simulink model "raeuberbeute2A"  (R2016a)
settings: Solver=ode45  StartTime=0.0  StopTime=250  FixedStep=0.1  MaxStep=1  RelTol=1e-3
undefined symbols (not defined in the file or in its folder): k, m0
libraries: simulink x1

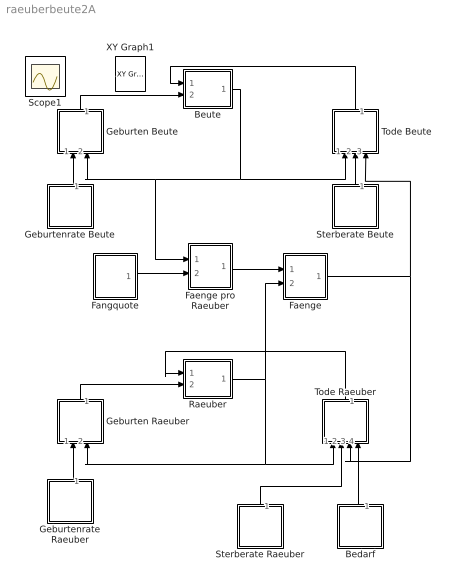
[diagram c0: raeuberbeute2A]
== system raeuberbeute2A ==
  Bedarf : Subsystem
  Beute : Subsystem
  Faenge : Subsystem
  Faenge pro Raeuber : Subsystem
  Fangquote : Subsystem
  Geburten Beute : Subsystem
  Geburten Raeuber : Subsystem
  Geburtenrate Beute : Subsystem
  Geburtenrate Raeuber : Subsystem
  Raeuber : Subsystem
  Sterberate Beute : Subsystem
  Sterberate Raeuber : Subsystem
  Tode Beute : Subsystem
  Tode Raeuber : Subsystem
  Scope1 : Scope
  XY Graph1 : simulink/Sinks/XY Graph  IOType=viewer  SystemSampleTime=-1  xmin=0  xmax=30  ymin=0  ymax=60  st=-1
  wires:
  Beute/1(Out1) -> Tode Beute/1(In1), Geburten Beute/2(In2), Faenge pro Raeuber/1(In1)
  Faenge/1(Out1) -> Tode Beute/3(In3), Tode Raeuber/3(In3)
  Raeuber/1(Out1) -> Geburten Raeuber/2(In2), Tode Raeuber/1(In1), Faenge/2(In2)
  Fangquote/1(Out1) -> Faenge pro Raeuber/2(In2)
  Geburten Beute/1(Out1) -> Beute/2(In2)
  Geburtenrate Beute/1(Out1) -> Geburten Beute/1(In1)
  Tode Beute/1(Out1) -> Beute/1(In1)
  Sterberate Beute/1(Out1) -> Tode Beute/2(In2)
  Geburten Raeuber/1(Out1) -> Raeuber/2(In2)
  Geburtenrate Raeuber/1(Out1) -> Geburten Raeuber/1(In1)
  Tode Raeuber/1(Out1) -> Raeuber/1(In1)
  Bedarf/1(Out1) -> Tode Raeuber/4(In4)
  Sterberate Raeuber/1(Out1) -> Tode Raeuber/2(In2)
  Faenge pro Raeuber/1(Out1) -> Faenge/1(In1)

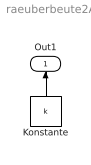
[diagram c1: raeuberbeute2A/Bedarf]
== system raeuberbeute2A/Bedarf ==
  Konstante : Constant  Value=k
  Out1 : Outport
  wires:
  Konstante/1 -> Out1/1

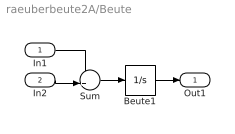
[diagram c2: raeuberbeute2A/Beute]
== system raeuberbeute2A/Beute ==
  In1 : Inport
  In2 : Inport  Port=2
  Beute1 : Integrator  InitialCondition=m0
  Sum : Sum  Inputs=-+|
  Out1 : Outport
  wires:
  In2/1 -> Sum/2
  Beute1/1 -> Out1/1
  In1/1 -> Sum/1
  Sum/1 -> Beute1/1

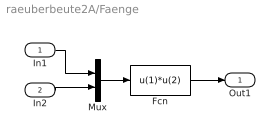
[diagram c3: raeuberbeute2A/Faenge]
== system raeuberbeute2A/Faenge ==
  In1 : Inport
  In2 : Inport  Port=2
  Fcn : Fcn  Expr=u(1)*u(2)
  Mux : Mux  Inputs=2
  Out1 : Outport
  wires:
  In2/1 -> Mux/2
  In1/1 -> Mux/1
  Mux/1 -> Fcn/1
  Fcn/1 -> Out1/1

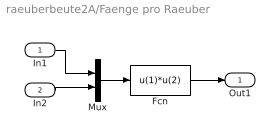
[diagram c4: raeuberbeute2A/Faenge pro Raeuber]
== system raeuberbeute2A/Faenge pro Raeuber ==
  In1 : Inport
  In2 : Inport  Port=2
  Fcn : Fcn  Expr=u(1)*u(2)
  Mux : Mux  Inputs=2
  Out1 : Outport
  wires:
  In2/1 -> Mux/2
  In1/1 -> Mux/1
  Mux/1 -> Fcn/1
  Fcn/1 -> Out1/1

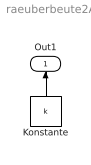
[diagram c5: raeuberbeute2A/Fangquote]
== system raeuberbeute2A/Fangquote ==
  Konstante : Constant  Value=k
  Out1 : Outport
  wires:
  Konstante/1 -> Out1/1

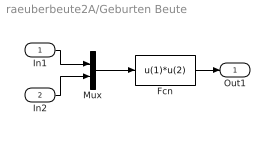
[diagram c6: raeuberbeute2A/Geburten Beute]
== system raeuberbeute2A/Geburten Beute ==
  In1 : Inport
  In2 : Inport  Port=2
  Fcn : Fcn  Expr=u(1)*u(2)
  Mux : Mux  Inputs=2
  Out1 : Outport
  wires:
  In2/1 -> Mux/2
  In1/1 -> Mux/1
  Mux/1 -> Fcn/1
  Fcn/1 -> Out1/1

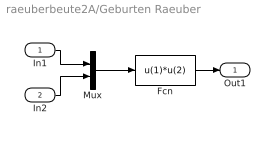
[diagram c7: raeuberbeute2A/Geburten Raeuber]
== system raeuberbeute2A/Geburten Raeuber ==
  In1 : Inport
  In2 : Inport  Port=2
  Fcn : Fcn  Expr=u(1)*u(2)
  Mux : Mux  Inputs=2
  Out1 : Outport
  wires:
  In2/1 -> Mux/2
  In1/1 -> Mux/1
  Mux/1 -> Fcn/1
  Fcn/1 -> Out1/1

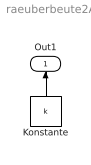
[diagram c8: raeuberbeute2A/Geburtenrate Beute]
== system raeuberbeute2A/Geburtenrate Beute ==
  Konstante : Constant  Value=k
  Out1 : Outport
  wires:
  Konstante/1 -> Out1/1

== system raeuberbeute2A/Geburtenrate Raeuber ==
  Konstante : Constant  Value=k
  Out1 : Outport
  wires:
  Konstante/1 -> Out1/1

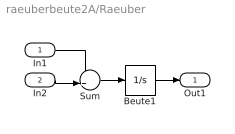
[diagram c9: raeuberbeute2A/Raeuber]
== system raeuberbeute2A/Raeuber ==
  In1 : Inport
  In2 : Inport  Port=2
  Beute1 : Integrator  InitialCondition=m0
  Sum : Sum  Inputs=-+|
  Out1 : Outport
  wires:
  In2/1 -> Sum/2
  Beute1/1 -> Out1/1
  In1/1 -> Sum/1
  Sum/1 -> Beute1/1

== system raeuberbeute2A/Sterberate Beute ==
  Konstante : Constant  Value=k
  Out1 : Outport
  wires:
  Konstante/1 -> Out1/1

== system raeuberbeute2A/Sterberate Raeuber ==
  Konstante : Constant  Value=k
  Out1 : Outport
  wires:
  Konstante/1 -> Out1/1

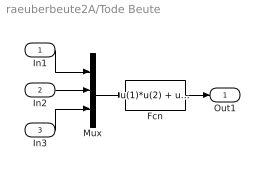
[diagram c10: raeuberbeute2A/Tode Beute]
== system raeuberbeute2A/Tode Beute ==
  In1 : Inport
  In2 : Inport  Port=2
  In3 : Inport  Port=3
  Fcn : Fcn  Expr=u(1)*u(2) + u(3)
  Mux : Mux  Inputs=3
  Out1 : Outport
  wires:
  In2/1 -> Mux/2
  In1/1 -> Mux/1
  Mux/1 -> Fcn/1
  Fcn/1 -> Out1/1
  In3/1 -> Mux/3

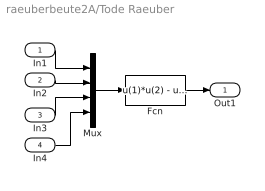
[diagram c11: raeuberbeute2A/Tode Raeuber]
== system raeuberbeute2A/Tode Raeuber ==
  In1 : Inport
  In2 : Inport  Port=2
  In3 : Inport  Port=3
  In4 : Inport  Port=4
  Fcn : Fcn  Expr=u(1)*u(2) - u(3)/u(4)
  Mux : Mux
  Out1 : Outport
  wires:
  In2/1 -> Mux/2
  In1/1 -> Mux/1
  Mux/1 -> Fcn/1
  Fcn/1 -> Out1/1
  In3/1 -> Mux/3
  In4/1 -> Mux/4
